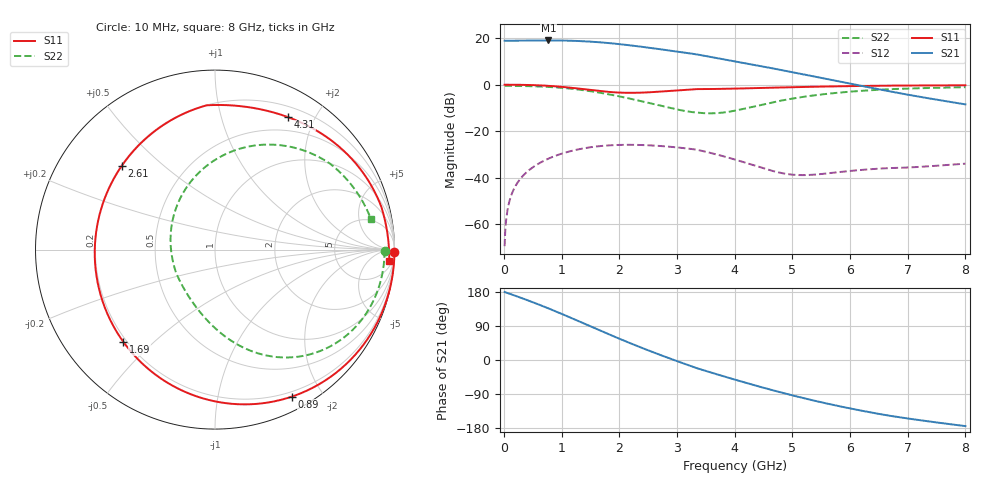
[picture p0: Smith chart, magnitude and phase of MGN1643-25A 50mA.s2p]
! Port[1] = GATE
! Port[2] = DRAIN
! [Type]  S-parameter s2p file touchstone ver. 1.0
! [Object]  MGN1643-25A
! [Bias]  50 mA
! [Version]  1.0
! [Date]  Tue May 19 13:03:48 2026
! [Source]  This file was created in JSC "ICC Milandr".
! [Disclaimer] Property of JSC "ICC Milandr". Unauthorized reproduction and/or distribution is strictly prohibited.
!  The file and the data are provided "AS IS" and with all faults and disclaim all warranties, express and implied, including
!  without limitation any implied warranties of merchantability, fitness for a particular purpose.
!  JSC "ICC Milandr" assumes no liability for:
!  1) the accuracy of the data provided;
!  2) the proper functioning of this data;
!  3) infringement of patents, copyrights or intellectual property rights resulting from the use of this data.
!  JSC "ICC Milandr" reserves the right to make changes to the products and the data without prior notice.
!  Please, be aware that your receipt and use of the file provided shall serve as acceptance of these terms and conditions.
!  If you do not accept these terms, you should return or destroy this file and any other accompanying information immediately.
# Hz S MA R 12.5
! freq  S11mag  S11ang  S21mag  S21ang  S12mag  S12ang  S22mag  S22ang
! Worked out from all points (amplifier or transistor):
!   800 points, 10 MHz to 8 GHz, reference 12.5 ohm
!   highest |S21| = 19.0 dB at 770 MHz (marker M1)
!   |S21| within 3 dB of that: start of sweep to 2.475 GHz
!   unconditionally stable (mu >= 1): 3.454 GHz to 7.532 GHz
!   at 1.34 GHz: K = 0.40, MSG = 23.1 dB, |S12| = -27.5 dB
!   at 4.01 GHz: K = 1.71, MAG = 16.2 dB, |S12| = -32.2 dB
!   at 8 GHz: K = 0.81, MSG = 12.7 dB, |S12| = -33.9 dB
!   S11 on the Smith chart (normalised r, x): 10 MHz: open; 890 MHz: 0.15, -1.65; 1.69 GHz: 0.19, -0.40; 2.61 GHz: 0.20, +0.37; 4.31 GHz: 0.32, +1.65; 8 GHz: 11, -26
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1e7  0.9999 -0.6  8.839 179.4  0.0003386 83.0  0.9449 -0.3
9e7  0.9998 -5.9  8.83 175.2  0.003017 84.9  0.9447 -3.1
2e8  0.9981 -13.1  8.843 169.3  0.00671 80.0  0.9429 -7.0
4.9e8  0.9824 -32.7  8.906 153.0  0.01648 65.5  0.9287 -17.3
7.7e8  0.9467 -53.0  8.945 136.2  0.02578 50.3  0.8981 -27.7
8.9e8  0.9246 -62.3  8.936 128.7  0.02962 43.6  0.8789 -32.3
1.13e9  0.8692 -82.1  8.839 113.3  0.03673 29.5  0.8292 -41.6
1.35e9  0.8104 -101.7  8.639 98.8  0.04226 16.4  0.7709 -50.1
1.69e9  0.7246 -134.9  8.113 76.2  0.04828 -4.1  0.6644 -63.1
1.92e9  0.6855 -158.4  7.638 61.3  0.05044 -17.7  0.5877 -71.7
2.14e9  0.6698 179.5  7.132 47.3  0.05115 -30.4  0.5159 -79.9
2.37e9  0.6753 157.9  6.583 33.2  0.05067 -43.1  0.4457 -88.8
2.61e9  0.6986 137.9  6.018 19.1  0.04913 -55.9  0.3799 -99.2
2.68e9  0.7076 132.6  5.857 15.0  0.04851 -59.6  0.3623 -102.6
3.01e9  0.7561 110.8  5.14 -3.5  0.04484 -76.4  0.2922 -122.0
3.33e9  0.8038 93.8  4.511 -20.9  0.04035 -92.2  0.253 -148.4
4.01e9  0.8258 69.6  3.177 -52.1  0.02453 -107.0  0.2779 150.1
4.31e9  0.8427 61.1  2.713 -65.2  0.01886 -107.9  0.3355 127.1
4.81e9  0.8735 48.9  2.067 -85.9  0.01265 -96.7  0.4565 98.1
5.34e9  0.9038 37.6  1.534 -105.9  0.01159 -74.9  0.5825 75.5
6.67e9  0.9569 14.5  0.7272 -146.8  0.01613 -64.9  0.8004 36.7
8e9  0.9727 -3.7  0.3784 -174.4  0.0201 -85.6  0.8855 11.1
